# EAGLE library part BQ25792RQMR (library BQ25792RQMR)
BQ25792 I 2C Controlled, 1-4 Cell, 5-A Buck-Boost Battery Charger with Dual-Input Selector and USB PD 3.0 OTG Output Source: Datasheet
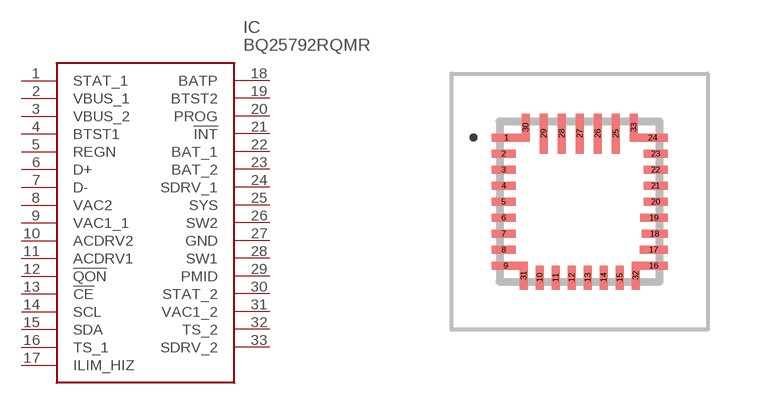
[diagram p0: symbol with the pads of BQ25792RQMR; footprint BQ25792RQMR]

Designator prefix IC

## BQ25792RQMR (Arrow_Part_Number: BQ25792RQMR; Arrow_Price-Stock: https://www.arrow.com/en/products/bq25792rqmr/texas-instruments?region=nac; Description: BQ25792 I 2C Controlled, 1-4 Cell, 5-A Buck-Boost Battery Charger with Dual-Input Selector and USB PD 3.0 OTG Output; Height: 1mm; Manufacturer_Name: Texas Instruments; Manufacturer_Part_Number: BQ25792RQMR; Mouser_Part_Number: 595-BQ25792RQMR; Mouser_Price-Stock: https://www.mouser.co.uk/ProductDetail/Texas-Instruments/BQ25792RQMR?qs=81r%252BiQLm7BSrfMJlEm4Auw%3D%3D)  [BQ25792RQMR]
1  STAT_1
2  VBUS_1
3  VBUS_2
4  BTST1
5  REGN
6  D+
7  D-
8  VAC2
9  VAC1_1
10  ACDRV2
11  ACDRV1
12  !QON
13  !CE
14  SCL
15  SDA
16  TS_1
17  ILIM_HIZ
18  BATP
19  BTST2
20  PROG
21  !INT
22  BAT_1
23  BAT_2
24  SDRV_1
25  SYS
26  SW2
27  GND
28  SW1
29  PMID
30  STAT_2
31  VAC1_2
32  TS_2
33  SDRV_2

## Footprint BQ25792RQMR (pad centres in mm)
RQM0029A
smd 0.75 x 0.2: 1 -1.825,1.6; 24 1.825,1.6
smd 0.6 x 0.2: 2 -1.9,1.2; 3 -1.9,0.8; 4 -1.9,0.4; 5 -1.9,0; 6 -1.9,-0.4; 7 -1.9,-0.8; 8 -1.9,-1.2; 20 1.9,0; 21 1.9,0.4; 22 1.9,0.8; 23 1.9,1.2
smd 0.7 x 0.2: 9 -1.85,-1.6; 16 1.853,-1.6; 17 1.85,-1.2
smd 0.2 x 0.6: 10 -1,-1.9; 11 -0.6,-1.9; 12 -0.2,-1.9; 13 0.2,-1.9; 14 0.6,-1.9; 15 1,-1.9
smd 0.65 x 0.2: 18 1.875,-0.8
smd 0.68 x 0.2: 19 1.86,-0.4
smd 0.2 x 1: 25 0.9,1.7; 26 0.45,1.7; 27 0,1.7; 28 -0.45,1.7; 29 -0.9,1.7
smd 0.2 x 0.7: 30 -1.35,1.85; 31 -1.4,-1.85; 32 1.4,-1.85; 33 1.35,1.85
